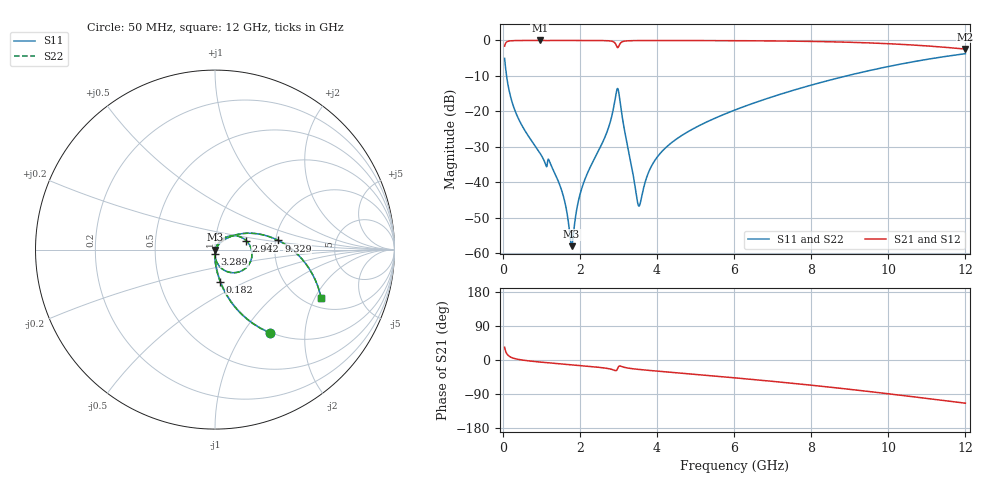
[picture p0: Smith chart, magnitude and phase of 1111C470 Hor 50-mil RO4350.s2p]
# GHz S MA R 50
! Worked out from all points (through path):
!   11951 points, 50 MHz to 12 GHz, reference 50 ohm
!   highest |S21| = -0.01 dB at 963 MHz (marker M1); lowest = -2.5 dB at 12 GHz (marker M2)
!   group delay of S21, straight-line fit = 26.7 ps
!   lowest |S11| = -58.1 dB at 1.788 GHz (marker M3), VSWR 1.00, Z = 50.1 - j0.0288 ohm
!   |S11| at or under -10 dB: 100.7 MHz to 8.923 GHz (8.822 GHz wide, 196 % of centre)
!   |S22| runs from -58.1 to -3.7 dB; largest |S21 - S12| = 0
!   S11 on the Smith chart (normalised r, x): 50 MHz: 0.99, -1.34; 182 MHz: 0.99, -0.37; 2.942 GHz: 1.41, +0.15; 3.289 GHz: 1.00, -0.05; 9.329 GHz: 2.07, +0.24; 12 GHz: 2.41, -2.25
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0.05  0.5581 -56.4  0.8296 33.6  0.8296 33.6  0.5581 -56.4
0.182  0.1804 -80.8  0.9832 9.1  0.9832 9.1  0.1804 -80.8
0.44  0.07259 -88.5  0.9967 1.0  0.9967 1.0  0.07259 -88.5
0.963  0.02585 -93.5  0.9987 -5.4  0.9987 -5.4  0.02585 -93.5
1.228  0.01872 -90.9  0.9975 -7.7  0.9975 -7.7  0.01872 -90.9
1.481  0.009098 -92.8  0.9987 -10.1  0.9987 -10.1  0.009098 -92.8
1.618  0.005072 -87.9  0.9987 -11.3  0.9987 -11.3  0.005072 -87.9
1.788  0.001248 -13.3  0.9986 -12.8  0.9986 -12.8  0.001248 -13.3
2.042  0.007878 64.4  0.9984 -15.0  0.9984 -15.0  0.007878 64.4
2.708  0.05152 59.5  0.9911 -22.1  0.9911 -22.1  0.05152 59.5
2.942  0.1807 16.2  0.8624 -28.1  0.8624 -28.1  0.1807 16.2
3.018  0.1742 -47.2  0.8465 -16.2  0.8465 -16.2  0.1742 -47.2
3.289  0.02377 -88.6  0.9901 -22.0  0.9901 -22.0  0.02377 -88.6
3.538  0.004598 -14.3  0.9953 -25.0  0.9953 -25.0  0.004598 -14.3
3.78  0.01363 48.6  0.9964 -27.3  0.9964 -27.3  0.01363 48.6
4.034  0.02356 53.5  0.9966 -29.6  0.9966 -29.6  0.02356 53.5
4.756  0.04965 51.2  0.996 -35.9  0.996 -35.9  0.04965 51.2
6.025  0.1044 41.4  0.9915 -47.1  0.9915 -47.1  0.1044 41.4
8.017  0.2352 22.5  0.9681 -66.6  0.9681 -66.6  0.2352 22.5
9.329  0.3567 8.2  0.9296 -81.1  0.9296 -81.1  0.3567 8.2
10.009  0.4289 0.2  0.8984 -89.2  0.8984 -89.2  0.4289 0.2
12  0.6496 -24.5  0.7541 -114.0  0.7541 -114.0  0.6496 -24.5
